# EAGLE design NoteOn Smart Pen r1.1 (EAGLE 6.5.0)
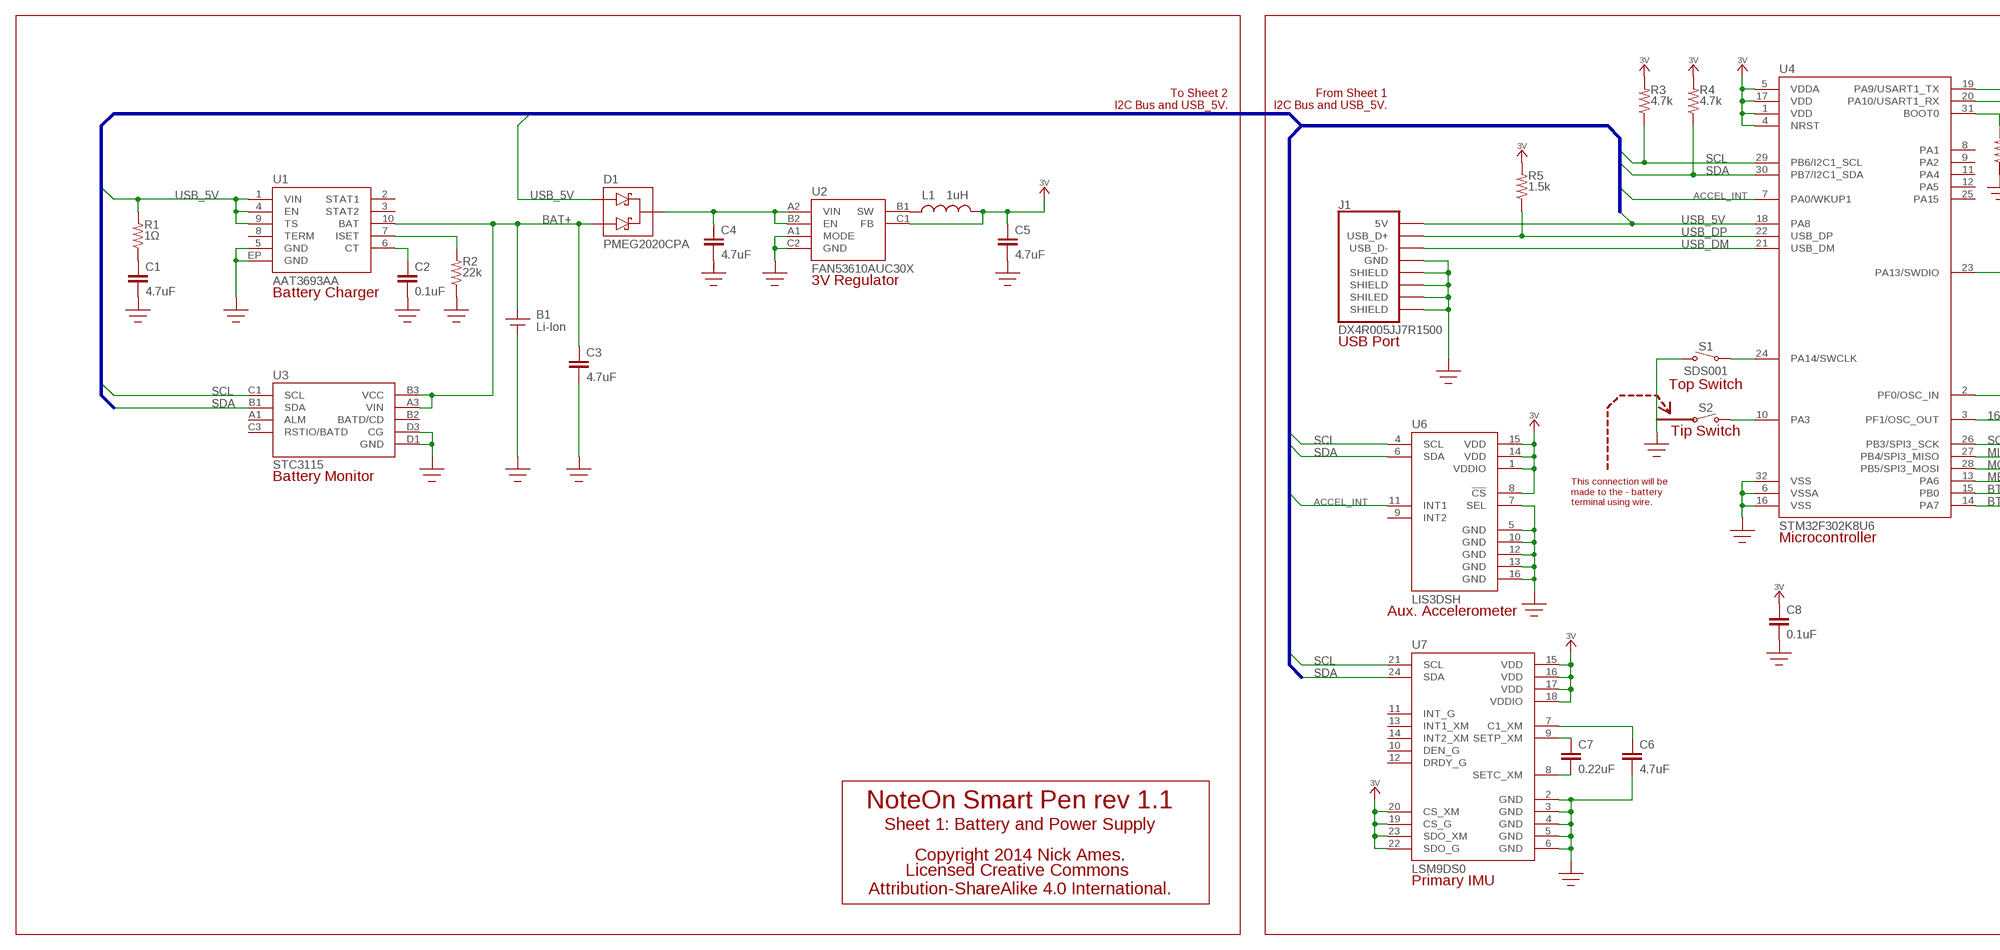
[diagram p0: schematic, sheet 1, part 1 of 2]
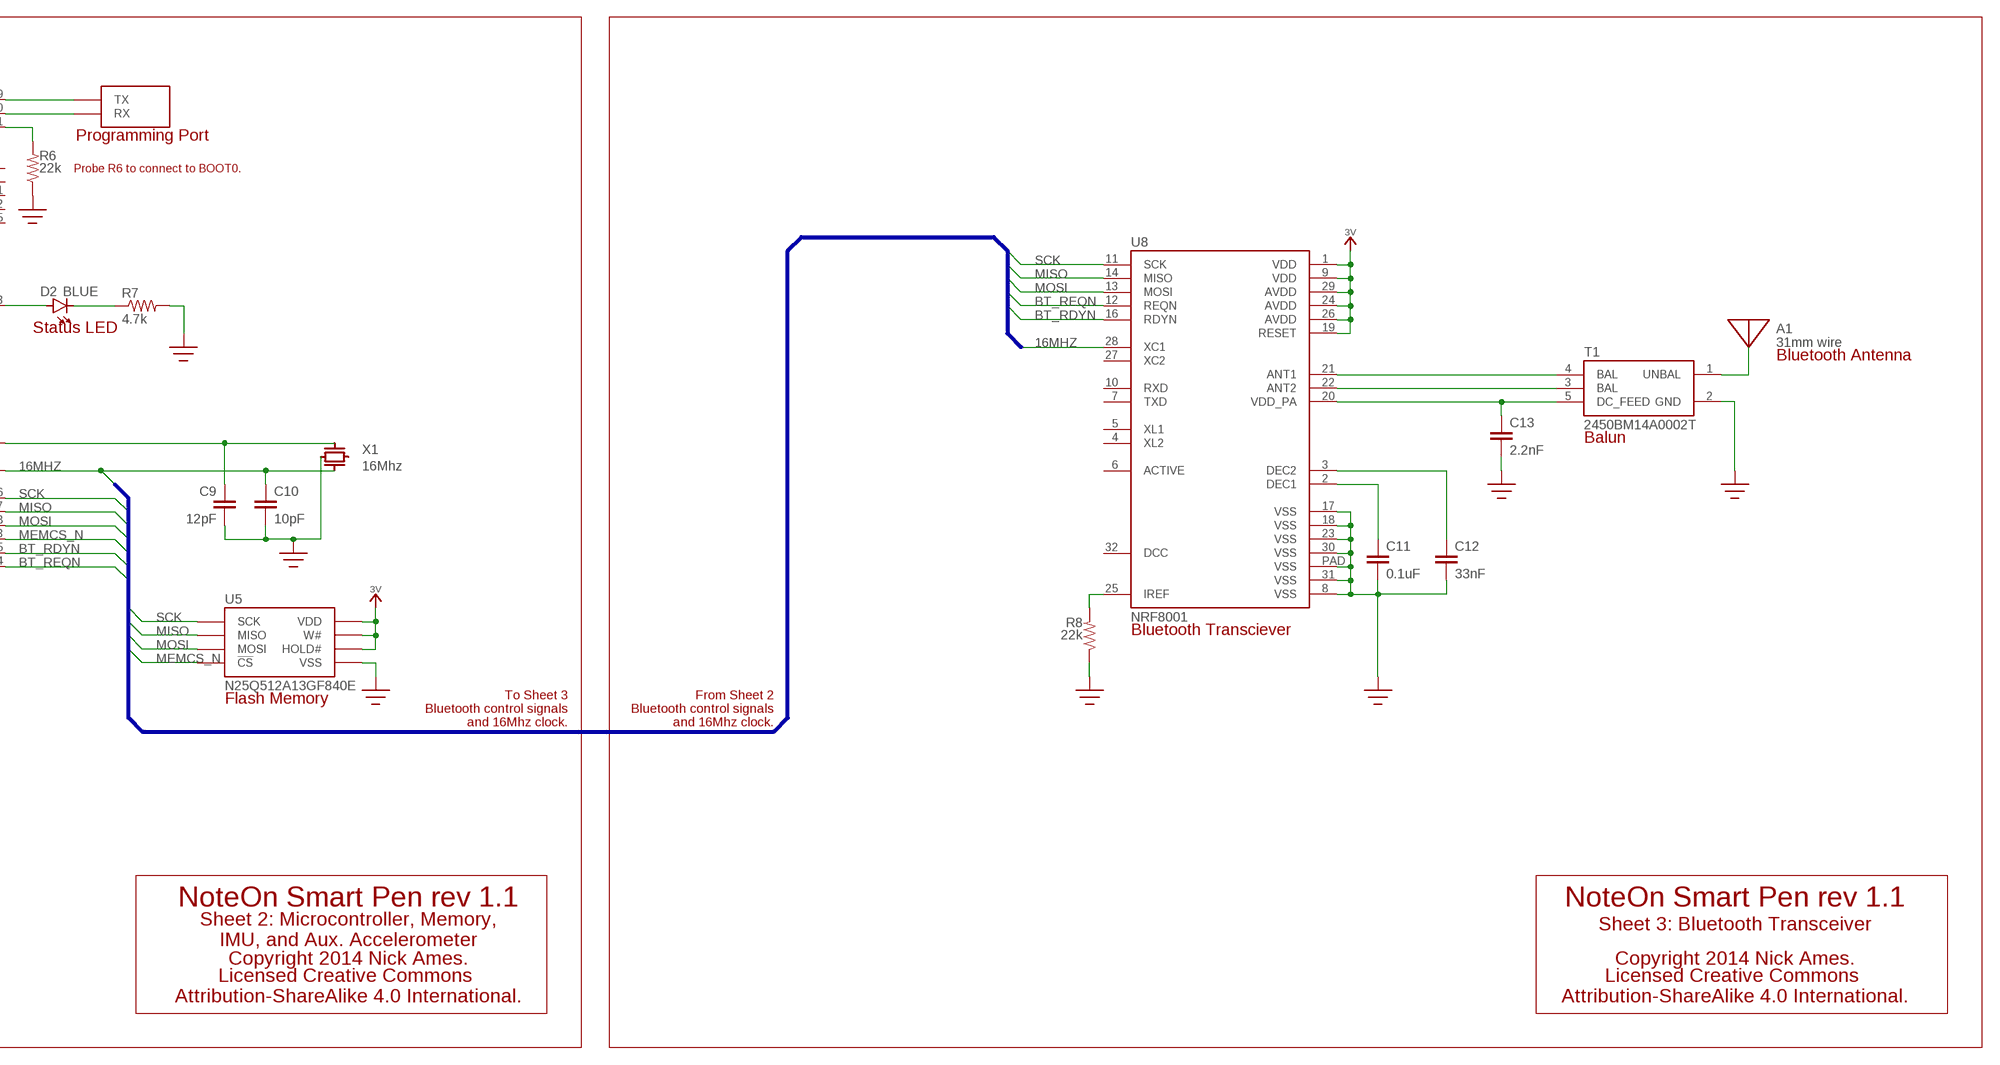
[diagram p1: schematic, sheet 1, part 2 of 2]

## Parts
A1  31mm wire  ANTENNA-WIRE  [WIRE-1]
B1  Li-Ion  BATTERY-1CELL  [BATTERY-WIRETERM]
C1  4.7uF  CAP402  [0402]
C2  0.1uF  CAP402  [0402]
C3  4.7uF  CAP402  [0402]
C4  4.7uF  CAP402  [0402]
C5  4.7uF  CAP402  [0402]
C6  4.7uF  CAP402  [0402]
C7  0.22uF  CAP402  [0402]
C8  0.1uF  CAP402  [0402]
C9  12pF  CAP402  [0402]
C10  10pF  CAP402  [0402]
C11  0.1uF  CAP402  [0402]
C12  33nF  CAP402  [0402]
C13  2.2nF  CAP402  [0402]
D1  PMEG2020CPA  [SOT1061]
D2  BLUE  LED0603  [LED-0603]
J1  DX4R005JJ7R1500  USB_CONNECTORMICRO-MID-SMD  [DX4R005JJ7R1500]
L1  1uH  INDUCTOR805  [0805-IND]
R1  1Ω  RESISTOR402  [0402]
R2  22k  RESISTOR402  [0402]
R3  4.7k  RESISTOR402  [0402]
R4  4.7k  RESISTOR402  [0402]
R5  1.5k  RESISTOR402  [0402]
R6  22k  RESISTOR402  [0402]
R7  4.7k  RESISTOR402  [0402]
R8  22k  RESISTOR402  [0402]
S1  SDS001  SWITCH-SPSTSDS001  [SDS001R]
S2  SWITCH-SPST-OFFBOARD  [TESTPOINT]
T1  2450BM14A0002T  [JOHNASON_BALUN]
U1  AAT3693AA  AAT3693  [TDFN-10]
U2  FAN53610AUC30X  FAN53600  [WLCSP-6]
U3  STC3115  [CSP-10]
U4  STM32F302K8U6  STM32F302K8U6QFN-32  [QFN-32-0.5]
U5  N25Q512A13GF840E  [V-PDFN-8]
U6  LIS3DSH  [LGA-16]
U7  LSM9DS0  [LGA-24]
U8  NRF8001  [QFN-32-0.5-EP]
U$20  STM-PROGPORT  [STM-PROGPORT]
X1  16Mhz  CRYSTAL-2GND  [TXC-8Y]

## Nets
3V: C5.1 C8.1 L1.P$2 R3.2 R4.2 R5.2 U2.C1(FB) U4.1(VDD) U4.4(NRST) U4.5(VDDA) U4.17(VDD) U5.3(W#) U5.7(HOLD#) U5.8(VDD) U6.1(VDDIO) U6.8(!CS!) U6.14(VDD) U6.15(VDD) U7.15(VDD) U7.16(VDD) U7.17(VDD) U7.18(VDDIO) U7.19(CS_G) U7.20(CS_XM) U7.22(SDO_G) U7.23(SDO_XM) U8.1(VDD) U8.9(VDD) U8.19(RESET) U8.24(AVDD) U8.26(AVDD) U8.29(AVDD)
16MHZ: C10.1 U4.3(PF1/OSC_OUT) U8.28(XC1) X1.X2(XTAL2)
ACCEL_INT: U4.7(PA0/WKUP1) U6.11(INT1)
BAT+: B1.+ C3.1 D1.A2 U1.10(BAT) U3.A3(VIN) U3.B3(VCC)
BOOT0: R6.2 U4.31(BOOT0)
BT_RDYN: U4.15(PB0) U8.16(RDYN)
BT_REQN: U4.14(PA7) U8.12(REQN)
GND: B1.- C1.2 C2.2 C3.2 C4.2 C5.2 C6.2 C8.2 C9.2 C10.2 C11.2 C12.2 C13.2 J1.5(GND) J1.SHIELD1(SHIELD) J1.SHIELD2(SHIELD) J1.SHIELD3(SHIELD) J1.SHIELD4(SHILED) R2.1 R6.1 R7.2 R8.1 S1.2 T1.2(GND) U1.5(GND) U1.EP(GND) U2.A1(MODE) U2.C2(GND) U3.D1(GND) U3.D3(CG) U4.6(VSSA) U4.16(VSS) U4.32(VSS) U5.4(VSS) U6.5(GND) U6.7(SEL) U6.10(GND) U6.12(GND) U6.13(GND) U6.16(GND) U7.2(GND) U7.3(GND) U7.4(GND) U7.5(GND) U7.6(GND) U8.8(VSS) U8.17(VSS) U8.18(VSS) U8.23(VSS) U8.30(VSS) U8.31(VSS) U8.PAD(VSS) X1.GND2(GND)
MEMCS_N: U4.13(PA6) U5.1(!CS!)
MISO: U4.27(PB4/SPI3_MISO) U5.2(MISO) U8.14(MISO)
MOSI: U4.28(PB5/SPI3_MOSI) U5.5(MOSI) U8.13(MOSI)
N$1: C1.1 R1.1
N$2: C9.1 U4.2(PF0/OSC_IN) X1.X1(XTAL1)
N$3: C2.1 U1.6(CT)
N$4: S1.1 U4.24(PA14/SWCLK)
N$5: D2.C R7.1
N$6: D2.A U4.23(PA13/SWDIO)
N$7: R2.2 U1.7(ISET)
N$8: L1.P$1 U2.B1(SW)
N$9: S2.1 U4.10(PA3)
N$10: R8.2 U8.25(IREF)
N$14: T1.4(BAL) U8.21(ANT1)
N$15: C7.1 U7.9(SETP_XM)
N$16: C7.2 U7.8(SETC_XM)
N$17: C6.1 U7.7(C1_XM)
N$18: T1.3(BAL) U8.22(ANT2)
N$19: C13.1 T1.5(DC_FEED) U8.20(VDD_PA)
N$20: C11.1 U8.2(DEC1)
N$21: C12.1 U8.3(DEC2)
N$22: A1.1(FEED) T1.1(UNBAL)
REG_VIN: C4.1 D1.C U2.A2(VIN) U2.B2(EN)
RX: U4.20(PA10/USART1_RX) U$20.RX
SCK: U4.26(PB3/SPI3_SCK) U5.6(SCK) U8.11(SCK)
SCL: R3.1 U3.C1(SCL) U4.29(PB6/I2C1_SCL) U6.4(SCL) U7.21(SCL)
SDA: R4.1 U3.B1(SDA) U4.30(PB7/I2C1_SDA) U6.6(SDA) U7.24(SDA)
TX: U4.19(PA9/USART1_TX) U$20.TX
USB_5V: D1.A1 J1.1(5V) R1.2 U1.1(VIN) U1.4(EN) U1.9(TS) U4.18(PA8)
USB_DM: J1.2(USB_D-) U4.21(USB_DM)
USB_DP: J1.3(USB_D+) R5.1 U4.22(USB_DP)
Unconnected: U1.2(STAT1) U1.3(STAT2) U1.8(TERM) U3.A1(ALM) U3.B2(BATD/CD) U3.C3(RSTIO/BATD) U4.8(PA1) U4.9(PA2) U4.11(PA4) U4.12(PA5) U4.25(PA15) U6.9(INT2) U7.10(DEN_G) U7.11(INT_G) U7.12(DRDY_G) U7.13(INT1_XM) U7.14(INT2_XM) U8.4(XL2) U8.5(XL1) U8.6(ACTIVE) U8.7(TXD) U8.10(RXD) U8.27(XC2) U8.32(DCC) X1.GND

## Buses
USB_5V,SDA,SCL,ACCEL_INT
SCK,MISO,MOSI,MEMCS_N,16MHZ,BT_REQN,BT_RDYN

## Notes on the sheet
- To Sheet 2
  I2C Bus and USB_5V.
- From Sheet 1
  I2C Bus and USB_5V.
- Programming Port
- Probe R6 to connect to BOOT0.
- 3V Regulator
- Battery Charger | Status LED
- Bluetooth Antenna
- USB Port
- Top Switch
- Balun
- Tip Switch
- Battery Monitor
- This connection will be
  made to the - battery 
  terminal using wire.
- Microcontroller
- Bluetooth Transciever
- Aux. Accelerometer
- To Sheet 3
  Bluetooth control signals
  and 16Mhz clock.
- From Sheet 2
  Bluetooth control signals
  and 16Mhz clock.
- Flash Memory
- NoteOn Smart Pen rev 1.1 | NoteOn Smart Pen rev 1.1 | NoteOn Smart Pen rev 1.1
- Sheet 1: Battery and Power Supply | Sheet 3: Bluetooth Transceiver
- Sheet 2: Microcontroller, Memory,
  IMU, and Aux. Accelerometer
- Copyright 2014 Nick Ames. | Copyright 2014 Nick Ames. | Copyright 2014 Nick Ames.
- Licensed Creative Commons 
  Attribution-ShareAlike 4.0 International.
- Licensed Creative Commons 
  Attribution-ShareAlike 4.0 International.
- Licensed Creative Commons 
  Attribution-ShareAlike 4.0 International.
- Primary IMU

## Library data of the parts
A1 = NA-lib:ANTENNA-WIRE
B1 = NA-lib:BATTERY-1CELL
C1-C13 = NA-lib:CAP: Capacitor
D1 = NA-lib:PMEG2020CPA
D2 = NA-lib:LED: LEDs
J1 = NA-lib:USB_CONNECTOR
L1 = NA-lib:INDUCTOR: Inductors
R1-R8 = NA-lib:RESISTOR: Resistor
S1 = NA-lib:SWITCH-SPST
S2 = NA-lib:SWITCH-SPST-OFFBOARD
T1 = NA-lib:2450BM14A0002T
U1 = NA-lib:AAT3693
U2 = NA-lib:FAN53600
U3 = NA-lib:STC3115
U4 = NA-lib:STM32F302K8U6
U5 = NA-lib:N25Q512A13GF840E
U6 = NA-lib:LIS3DSH
U7 = NA-lib:LSM9DS0
U8 = NA-lib:NRF8001
U$20 = NA-lib:STM-PROGPORT
X1 = NA-lib:CRYSTAL-2GND

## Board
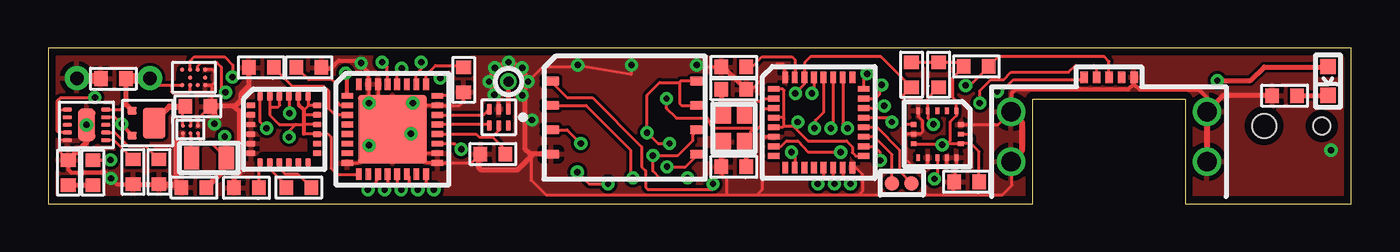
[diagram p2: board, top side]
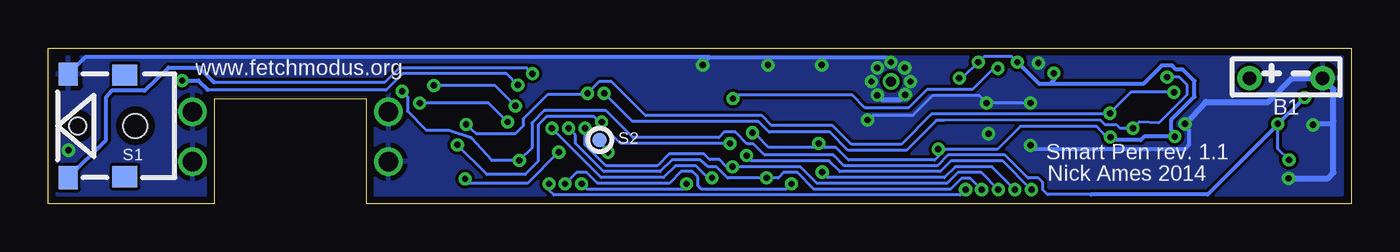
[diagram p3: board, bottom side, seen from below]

Size 67.87 x 8.13 mm. Coordinates in mm from the lower left corner, seen from the top.
Outline: 67.87,0 67.87,8.13 0,8.13 0,0 51.28,0 51.28,5.46 59.21,5.46 59.21,0 67.87,0
Copper layers (1*16): Top 0.0356mm / dielectric 1.5011mm / Bottom 0.0356mm
Design rules "LaenPCBOrder-tented_vias": minimum track width 6mil, minimum drill 13mil, track to track 6mil, track to pad 6mil, pad to pad 6mil, via to via 6mil, smd to smd 6mil, copper to edge 15mil, drill to drill 6mil, minimum pad ring 7mil, minimum via ring 7mil, stop-mask expansion 3mil, vias tented up to drill 25mil, thermal gap 10mil
tRestrict: area 16,3.7 to 16.1,4.1; area 19.7,3.7 to 19.8,4.1; area 11.1,2.5 to 13.7,2.5; area 13.6,2.5 to 13.7,3.4; area 1.4,3.9 to 1.5,4.3; area 2.5,3.9 to 2.6,4.4; area 6.8,6.4 to 7.2,6.8

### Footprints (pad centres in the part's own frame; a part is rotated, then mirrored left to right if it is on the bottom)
WIRE-1 = drill 0.508: 1 0,0
BATTERY-WIRETERM = drill 0.7 pad 1.27: + -1.905,0; - 1.905,0
0402 = smd 0.7 x 0.762: 1 -0.65,0; 2 0.65,0
SOT1061 = smd 0.4 x 0.5: A1 -0.65,0.8; A2 0.65,0.8 | smd 1.6 x 1.2: C 0,-0.35
LED-0603 = smd 0.8 x 0.8: A -0.75,0; C 0.75,0
DX4R005JJ7R1500 = smd 0.4 x 0.6: 1 -1.3,6.096; 2 -0.65,6.096; 3 0,6.096; 4 0.65,6.096; 5 1.3,6.096 | drill 1 pad 1.422: SHIELD1 -5.1,1.7; SHIELD2 -5.1,4.3; SHIELD3 5.1,4.3; SHIELD4 5.1,1.7
0805-IND = smd 0.8 x 1.2: P$1 -0.9,0; P$2 0.9,0
SDS001R = smd 1 x 1.2: 1 1.95,2.7; 2 1.95,-2.7 | smd 1.3 x 1.1: NC -1,2.65; NC2 -1,-2.65 | hole 0.9: 1.45,0 | hole 1.25: -1.55,0
TESTPOINT = smd 0.762 x 0.762: 1 0,0
JOHNASON_BALUN = smd 0.25 x 0.55: 1 0.5,0.425; 2 0,0.425; 3 -0.5,0.425; 4 -0.5,-0.425; 5 0,-0.425; 6 0.5,-0.425
TDFN-10 = smd 0.5 x 0.2: 1 -1,0.8; 2 -1,0.4; 3 -1,0; 4 -1,-0.4; 5 -1,-0.8; 6 1,-0.8; 7 1,-0.4; 8 1,0; 9 1,0.4; 10 1,0.8 | smd 0.9 x 1.7: EP 0,0
WLCSP-6 = smd 0.2 x 0.2: A1 -0.2,0.4; A2 0.2,0.4; B1 -0.2,0; B2 0.2,0; C1 -0.2,-0.4; C2 0.2,-0.4
CSP-10 = smd 0.24 x 0.24: A1 0.4,0.6; A3 -0.4,0.6; B1 0.4,0.2; B2 0,0.2; B3 -0.4,0.2; C1 0.4,-0.2; C3 -0.4,-0.2; D1 0.4,-0.6; D2 0,-0.6; D3 -0.4,-0.6
QFN-32-0.5 = smd 0.6 x 0.3: 1 -2.35,1.75; 2 -2.35,1.25; 3 -2.35,0.75; 4 -2.35,0.25; 5 -2.35,-0.25; 6 -2.35,-0.75; 7 -2.35,-1.25; 8 -2.35,-1.75; 17 2.35,-1.75; 18 2.35,-1.25; 19 2.35,-0.75; 20 2.35,-0.25; 21 2.35,0.25; 22 2.35,0.75; 23 2.35,1.25; 24 2.35,1.75 | smd 0.3 x 0.6: 9 -1.75,-2.35; 10 -1.25,-2.35; 11 -0.75,-2.35; 12 -0.25,-2.35; 13 0.25,-2.35; 14 0.75,-2.35; 15 1.25,-2.35; 16 1.75,-2.35; 25 1.75,2.35; 26 1.25,2.35; 27 0.75,2.35; 28 0.25,2.35; 29 -0.25,2.35; 30 -0.75,2.35; 31 -1.25,2.35; 32 -1.75,2.35
V-PDFN-8 = smd 0.889 x 0.457: 1 -3.835,1.905; 2 -3.835,0.635; 3 -3.835,-0.635; 4 -3.835,-1.905; 5 3.835,-1.905; 6 3.835,-0.635; 7 3.835,0.635; 8 3.835,1.905
LGA-16 = smd 0.356 x 0.254: 1 -1.219,0.996; 2 -1.219,0.498; 3 -1.219,0; 4 -1.219,-0.498; 5 -1.219,-0.996; 9 1.219,-0.996; 10 1.219,-0.498; 11 1.219,0; 12 1.219,0.498; 13 1.219,0.996 | smd 0.254 x 0.356: 6 -0.5,-1.225; 7 0,-1.225; 8 0.5,-1.225; 14 0.5,1.225; 15 0,1.225; 16 -0.5,1.225
LGA-24 = smd 0.45 x 0.3: 1 -1.725,1.25; 2 -1.725,0.75; 3 -1.725,0.25; 4 -1.725,-0.25; 5 -1.725,-0.75; 6 -1.725,-1.25; 13 1.725,-1.25; 14 1.725,-0.75; 15 1.725,-0.25; 16 1.725,0.25; 17 1.725,0.75; 18 1.725,1.25 | smd 0.3 x 0.45: 7 -1.25,-1.725; 8 -0.75,-1.725; 9 -0.25,-1.725; 10 0.25,-1.725; 11 0.75,-1.725; 12 1.25,-1.725; 19 1.25,1.725; 20 0.75,1.725; 21 0.25,1.725; 22 -0.25,1.725; 23 -0.75,1.725; 24 -1.25,1.725
QFN-32-0.5-EP = smd 0.6 x 0.3: 1 -2.35,1.75; 2 -2.35,1.25; 3 -2.35,0.75; 4 -2.35,0.25; 5 -2.35,-0.25; 6 -2.35,-0.75; 7 -2.35,-1.25; 8 -2.35,-1.75; 17 2.35,-1.75; 18 2.35,-1.25; 19 2.35,-0.75; 20 2.35,-0.25; 21 2.35,0.25; 22 2.35,0.75; 23 2.35,1.25; 24 2.35,1.75 | smd 0.3 x 0.6: 9 -1.75,-2.35; 10 -1.25,-2.35; 11 -0.75,-2.35; 12 -0.25,-2.35; 13 0.25,-2.35; 14 0.75,-2.35; 15 1.25,-2.35; 16 1.75,-2.35; 25 1.75,2.35; 26 1.25,2.35; 27 0.75,2.35; 28 0.25,2.35; 29 -0.25,2.35; 30 -0.75,2.35; 31 -1.25,2.35; 32 -1.75,2.35 | smd 3.581 x 3.581: PAD 0,0
STM-PROGPORT = smd 0.762 x 0.762: RX 0,0; TX 0,1.016
TXC-8Y = smd 0.9 x 0.8: GND -0.7,0.55; GND2 0.7,-0.55; X1 -0.7,-0.55; X2 0.7,0.55

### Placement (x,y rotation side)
A1  23.98,6.38 0 top
B1  3.4,6.55 0 bottom
C1  1.05,1.63 90 top
C2  4.43,1.66 270 top
C3  3.4,6.53 180 top
C4  7.8,5.08 0 top
C5  7.61,0.85 180 top
C6  10.34,0.84 180 top
C7  13.06,0.85 180 top
C8  47.83,1.14 180 top
C9  35.71,5.97 0 top
C10  35.71,1.93 180 top
C11  13.59,7.11 0 top
C12  11.1,7.11 180 top
C13  23.16,2.59 180 top
D1  5.18,4.2 90 top
D2  66.65,6.4 270 top
J1  55.24,0.5 0 top
L1  8.38,2.39 0 top
R1  2.34,1.63 90 top
R2  5.78,1.66 90 top
R3  46.38,6.73 90 top
R4  44.96,6.73 90 top
R5  48.34,7.16 180 top
R6  35.71,7.14 0 top
R7  64.39,5.64 180 top
R8  21.64,6.46 90 top
S1  64.87,4.06 180 bottom
S2  39.14,3.33 0 bottom
T1  23.47,4.51 0 top
U1  2.01,4.11 0 top
U2  7.42,3.87 90 top
U3  7.59,6.59 90 top
U4  40.13,4.24 0 top
U5  30.02,4.5 0 top
U6  46.3,3.63 270 top
U7  12.29,3.89 0 top
U8  17.93,3.89 0 top
U$20  44.96,1.07 90 top
X1  35.71,3.94 270 top

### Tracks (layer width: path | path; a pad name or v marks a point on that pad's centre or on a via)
3V  (via drill 0.33 pad 0.69)
  Top 0.152: U2.C1 7.82,3.44 8.03,3.23 8.44,3.23 9.1,2.57 L1.P$2 | U8.29 17.66,7.13 v17.4,7.39 | 19.15,6.27 19.15,6.76 19.43,7.04 v19.43,7.39 | 13.34,3.66 13.36,3.64 U7.15 14.58,3.64 14.73,3.48 14.73,1.85 15.06,1.52 16.17,1.52 U8.9 | 13.06,5.16 13.06,5.6 U7.20 | U7.19 13.54,5.08 | 13.54,5.08 13.34,4.88 | U7.18 13.59,5.14 13.54,5.08 | U7.17 13.42,4.64 13.34,4.72 | U7.16 13.36,4.14 13.34,4.12 | U7.23 11.54,5.12 | 11.54,5.12 11.61,5.05 11.99,5.05 12.06,5.13 12.06,5.59 U7.22 | 11.54,5.12 11.54,4.64 12.04,4.14 12.9,4.14 | 12.9,4.14 13.26,4.14 13.34,4.06 | v20.42,6.55 20.7,6.55 20.93,6.33 20.93,5.71 20.85,5.64 U8.24 | v12.55,3.48 12.55,3.79 12.9,4.14 | U8.19 21.15,3.14 v21.51,2.85 | U5.8 32.94,6.4 32.89,6.35 | 32.89,6.35 32.89,5.23 32.99,5.13 U5.7 | 32.89,6.35 32.87,6.33 31.85,6.33 31.19,5.66 v31.19,3.71 31.75,3.15 v32.36,3.15 | U5.3 27.03,3.86 v27.74,3.15 | U4.5 38.26,3.99 38.33,4.06 | 38.33,4.06 38.33,4.45 | 38.33,4.45 38.28,4.5 U4.4 | 38.33,4.45 38.33,5.92 38.25,5.99 U4.1 | U4.17 42.06,2.49 41.88,2.67 41.88,2.97 41.58,3.28 39.57,3.28 38.79,4.06 | 38.33,4.06 38.79,4.06 | R4.2 R3.2 47.47,7.38 R5.2 47.12,6.59 47.12,5.54 47.3,5.35 U6.1 47.3,4.6 46.97,4.27 46.97,3.28 46.84,3.15 | 38.79,4.06 38.84,4.06 v39.04,4.27 | U6.15 47.9,3.63 48.08,3.45 48.08,3.28 48.01,3.2 | 48.01,3.2 47.95,3.15 47.55,3.15 U6.14 47.51,3.15 46.84,3.15 | U6.8 46.5,3.13 v46.56,3.07 46.76,3.07 46.84,3.15 | C8.1 48.48,2.73 48.01,3.2
  Top 0.203: 13.34,3.66 13.34,4.06 13.34,4.12 13.34,4.72 13.34,4.88 13.06,5.16 | U8.1 15.58,6.72 v15.49,6.81
  Top 0.254: 19.15,6.27 U8.26
  Top 0.305: C5.1 9.1,1.69 9.1,2.57 | 9.3,2.4 L1.P$2 9.28,3.42 v9.2,3.5
  Bottom 0.152: v20.42,6.55 20.3,6.55 v19.43,7.39 19.15,7.67 17.68,7.67 v17.4,7.39 | v12.55,3.48 12.75,3.48 13.26,4.04 17.25,4.04 18.44,2.85 21.13,2.85 | v21.51,2.85 21.13,2.85 | 21.13,2.85 21.69,2.29 26.19,2.29 26.85,2.95 27.61,2.95 27.61,3.02 v27.74,3.15 27.74,3.1 27.89,2.95 30.35,2.95 30.94,3.53 31.19,3.53 v31.19,3.71 | v32.36,3.15 38.05,3.15 39.12,4.22 | 39.12,4.22 39.45,4.55 41.91,4.55 42.34,4.12 42.34,2.21 43.03,1.52 45.01,1.52 v46.56,3.07 | v39.04,4.27 39.06,4.27 39.12,4.22
  Bottom 0.203: v12.55,3.48 12.39,3.33 10.97,3.33 10.79,3.5 v9.2,3.5 9.2,3.66 9.37,3.83 9.37,4.39 8.18,5.59 8.18,6.4 8.79,7.01 9.14,7.01 9.35,7.21 9.88,7.21 10.85,6.25 15.7,6.25 | 15.7,6.25 16.26,6.25 v17.4,7.39 | v15.49,6.81 15.49,6.45 15.7,6.25
16MHZ  (via drill 0.33 pad 0.69)
  Top 0.152: 36.56,3.24 X1.X2 36.55,3.52 36.55,3.73 36.75,3.94 | U8.28 18.18,6.88 v18.41,7.06 | 36.75,3.94 34.62,3.94 34.34,4.47 32.72,4.47 32.21,4.98 v32.21,5.49 | 36.75,3.94 36.96,3.94 37.11,4.09 37.11,4.83 37.26,4.98 37.77,4.98 U4.3
  Top 0.254: C10.1 36.36,3.14 X1.X2
  Bottom 0.152: v18.41,7.06 18.64,7.06 19.74,5.97 22.1,5.97 23.06,5 25.32,5 25.98,5.66 32.03,5.66 v32.21,5.49
ACCEL_INT  (via drill 0.33 pad 0.69)
  Top 0.152: U4.7 38.17,2.99 38.46,3.28 39.04,3.28 39.57,2.69 v41.27,2.69 | U6.11 46.3,1.45 v46.15,1.29
  Bottom 0.152: v41.27,2.69 42.9,1.07 45.92,1.07 v46.15,1.29
BAT+
  Top 0.152: U1.10 3.77,4.93 4.05,5.21 | B1.+ 5.67,6.19 6.44,6.19 | 6.44,6.19 U3.A3 | 6.44,6.19 6.44,5.83 6.5,5.77 7.29,5.77 7.39,5.87 U3.B3
  Top 0.254: C3.1 4.05,5.21 D1.A2
  Top 0.61: C3.1 B1.+
BOOT0
  Top 0.152: R6.2 36.65,7.14 37.19,7.67 38.73,7.67 38.89,7.52 U4.31
BT_RDYN  (via drill 0.33 pad 0.69)
  Top 0.152: U8.16 19.68,1.15 v20.09,0.74 | U4.15 41.38,1.44 v41.78,1.04
  Bottom 0.152: v20.09,0.74 20.37,0.46 41.53,0.46 41.78,0.71 v41.78,1.04
BT_REQN  (via drill 0.33 pad 0.69)
  Top 0.152: U8.12 17.68,0.89 v17.53,0.74 | v27.56,1.65 28.17,1.04 v29.16,1.04 | U4.14 40.88,1.1 v40.95,1.04
  Bottom 0.152: v17.53,0.74 18.72,1.93 20.62,1.93 21.18,1.37 27.28,1.37 v27.56,1.65 | v29.16,1.04 29.44,0.76 33.86,0.76 34.04,0.94 34.04,1.4 34.31,1.68 34.9,1.68 35.51,1.07 39.27,1.07 39.83,1.63 40.36,1.63 v40.95,1.04
GND  (via drill 0.33 pad 0.69)
  Top 0.152: U1.5 0.61,3.33 0.56,3.28 0.56,2.77 C1.2 | U3.D3 8.53,6.19 | 8.53,6.19 8.71,6.38 8.71,6.83 8.55,6.99 U3.D1 | 8.53,6.19 8.53,5.26 C4.2 8.42,5.05 7.82,4.45 U2.C2 | U2.A1 7.02,3.38 6.96,3.33 6.76,3.33 6.66,3.23 | 8.66,4.8 8.66,4.75 8.76,4.65 | U7.2 10.56,4.65 9.98,4.65 | U7.4 10.55,3.66 9.98,3.66 | 10.55,3.15 U7.5 9.99,3.14 9.98,3.12 | U7.6 10.03,2.64 9.98,2.59 | U7.3 9.99,4.14 9.98,4.14 | U8.30 17.18,5.42 | U8.8 16.18,2.14 U8.PAD | 19.36,5.14 U8.23 21.42,5.14 21.64,5.36 R8.1 | U8.18 19.18,2.64 U8.PAD | U8.PAD 19.68,2.14 U8.17 22.06,2.14 22.4,2.48 C13.2 | 17.17,5.41 17.12,5.46 16.69,5.46 16.68,5.47 U8.31 16.68,6.84 | 14.29,7.06 C11.2 | 17.37,3.89 U8.PAD | 18.95,3.25 18.75,3.45 18.31,3.89 U8.PAD | v25.2,4.37 24.82,4.7 24.82,5.51 | T1.2 23.47,5.46 v23.24,5.69 | v16.31,7.34 16.24,7.28 | 25.15,2.59 25.15,1.25 25.93,0.46 35.38,0.46 | 35.38,0.46 36.91,0.46 | 36.91,0.46 42.22,0.46 | C10.2 35.06,1.56 35.33,1.29 35.33,0.51 35.38,0.46 | X1.GND2 35.16,3.54 35.31,3.54 | R6.1 33.88,7.14 v33.78,7.24 | U4.6 37.33,3.49 37.19,3.35 37.19,0.74 36.91,0.46 | 42.22,0.46 45.77,0.46 | 45.77,0.46 47.12,0.46 | 47.12,0.46 49.68,0.46 50.19,0.96 50.19,2.15 J1.SHIELD1 | 45.8,2.4 U6.10 45.81,2.14 45.57,1.91 | U6.13 47.3,2.04 47.22,1.91 | 47.22,1.91 46.89,1.91 46.79,2.01 46.8,2.02 U6.12 46.79,2.4 | 45.57,1.91 45.06,1.91 44.65,2.34 44.65,3.53 44.76,3.63 U6.7 45.41,3.63 45.52,3.73 45.52,4.34 45.31,4.55 U6.5 | U4.16 42.05,1.89 42.42,1.52 42.42,0.66 42.22,0.46 | C9.2 36.63,5.97 37.95,7.29 38.28,7.29 38.38,7.19 U4.32 | 47.22,1.91 47.22,1.18 C8.2 47.12,1.08 47.12,0.46 | 45.57,1.91 45.57,0.64 45.77,0.46 | U6.16 49.48,4.13 J1.SHIELD2 | v24.99,6.38 25.78,7.16 27.23,7.16 v27.58,7.24 30.38,6.76 v30.38,7.24
  Top 0.203: C1.2 1.05,1.79 1.22,1.63 2.97,1.63 v3.28,1.32 3.58,1.02 C2.2 | 14.29,7.06 14.73,7.06 15.14,7.47 16.05,7.47 16.24,7.28 16.68,6.84 | v16.71,3.05 18.09,3.05 v18.9,3.66 18.85,3.56 18.75,3.45 | J1.5 56.55,6.25 | 56.55,6.25 56.24,5.94 50.37,5.94 50.16,5.74 50.16,4.82 J1.SHIELD2 | 56.55,6.25 56.85,5.94 59.92,5.94 60.35,5.51 J1.SHIELD3
  Top 0.254: C2.2 R2.1 | U1.EP 2.01,4.52 1.96,4.57 | 6.66,3.23 6.66,1.15 C5.2 | C6.2 9.69,1.31 9.98,1.6 9.98,2.59 9.98,3.12 9.98,3.66 9.98,4.14 9.98,4.65 9.98,4.78 9.7,5.05 | 9.7,5.05 9.65,5.11 8.47,5.11 C4.2 | C12.2 10.45,6.13 10.03,5.71 10.03,5.38 9.7,5.05 | U8.30 | 17.18,5.42 17.17,5.41 17.17,4.65 U8.PAD 19.15,5.11 19.33,5.11 19.36,5.14 | U5.4 25.27,2.59 | 25.27,2.59 25.15,2.59 25.09,2.59 24.84,2.85 24.84,5.49 24.82,5.51 24.69,5.64 v24.69,5.66 v24.99,6.38 v24.69,7.09 v23.98,7.39 v23.27,7.09 v22.96,6.38 v23.24,5.69 | 22.4,2.48 22.4,1.93 22.55,1.78 24.46,1.78 25.27,2.59 | C10.2 35.06,3.14 X1.GND2 | R6.1 35.17,7.14 C9.2 36.26,5.84 | R7.2 61.18,5.64 J1.SHIELD3
  Top 0.305: C1.2 2.01,3.23 U1.EP | R2.1 6.79,1.01 C5.2 | 8.42,5.05 8.66,4.8 v8.66,4.17 | J1.SHIELD3 J1.SHIELD4 | J1.SHIELD2 50.16,4.8 50.7,4.27 50.7,2.75 J1.SHIELD1
  Top 0.61: C3.2 B1.-
  Bottom 0.152: 0.94,4.29 0.94,4.22 0.99,4.17 | v25.2,4.37 24.89,4.62 22.84,4.62 21.79,5.66 19.41,5.66 v19,5.26 v16.71,5.26 | v33.78,7.24 33.43,7.64
  Bottom 0.203: v8.66,4.17 8.66,4.06 8.46,3.86 8.46,3.07 8.69,2.85 16.51,2.85 v16.71,3.05 | v23.98,7.39 24.23,7.64 33.43,7.64 65.94,7.64 S1.2
  Bottom 0.254: 0.99,4.17 1.96,4.17 U1.EP | v23.24,5.69 23.52,5.41 24.43,5.41 v24.69,5.66
  Bottom 0.305: v3.28,1.32 1.25,1.32 0.94,1.63 0.94,4.29 0.94,5.97 B1.- 3.1,6.55 4.34,5.31 7.59,5.31 v8.66,4.17
  other vias: 2.01,4.11 66.8,2.79
  pour Top (isolate 0.152): 0.46,0.46 0.46,7.67 67.41,7.67 67.41,0.46
  pour Bottom (isolate 0.152): 0.46,0.46 0.46,7.67 67.41,7.67 67.41,0.46
MEMCS_N  (via drill 0.33 pad 0.69)
  Top 0.152: v34.62,1.04 34.62,0.76 31.22,0.76 31.11,0.86 31.11,1.73 30.91,1.93 30.91,2.97 28.35,5.54 27.03,5.54 26.19,6.38 U5.1 | U4.13 40.38,1.34 v40.08,1.04
  Bottom 0.152: v34.62,1.04 34.62,0.76 39.8,0.76 v40.08,1.04
MISO  (via drill 0.33 pad 0.69)
  Top 0.152: U8.14 18.8,1.42 18.8,1.14 19.2,0.74 v19.25,0.74 | U5.2 28.02,5.13 30.33,2.82 30.33,1.5 v30.45,1.35 | U4.27 40.88,4.1 v40.77,3.94
  Bottom 0.152: v19.25,0.74 19.84,1.32 20.32,1.32 20.88,0.76 27.99,0.76 28.85,1.63 29.57,1.63 29.84,1.35 v30.45,1.35 32.49,1.35 33.07,1.93 33.48,1.93 33.88,2.29 35.38,2.29 35.99,1.68 38.94,1.68 40.41,3.15 40.41,3.58 v40.77,3.94
MOSI  (via drill 0.33 pad 0.69)
  Top 0.152: U8.13 18.18,0.94 v18.39,0.74 | U4.28 40.38,4.77 39.95,4.34 39.95,4.17 v39.9,3.94 | v32.23,1.93 33.2,1.93 U5.5
  Bottom 0.152: v18.39,0.74 19.28,1.63 20.5,1.63 21.06,1.07 27.84,1.07 28.7,1.93 v32.23,1.93 32.54,1.93 32.92,2.31 33.43,2.31 33.71,2.59 35.53,2.59 36.14,1.98 38.81,1.98 39.9,3.07 v39.9,3.94
N$1
  Top 0.254: C1.1 R1.1
N$2
  Top 0.152: 35.06,4.8 35.06,4.59 | 35.06,5.28 35.09,5.36 37.11,5.36 37.24,5.49 U4.2
  Top 0.254: X1.X1 35.06,4.74 35.06,4.8 35.06,5.28 C9.1
N$3
  Top 0.152: C2.1 3.42,3.33 U1.6
N$4  (via drill 0.33 pad 0.69)
  Top 0.152: U4.24 42.48,6.62 v42.65,6.78
  Bottom 0.152: 59.21,6.33 50.34,6.33 49.58,7.09 42.95,7.09 v42.65,6.78
  Bottom 0.203: S1.1 64.85,3.34 64.85,5.56 64.54,5.89 62.84,5.89 61.59,7.11 59.99,7.11 59.21,6.33
N$5
  Top 0.254: R7.1 66.64,5.64 D2.C
N$6  (via drill 0.33 pad 0.69)
  Top 0.152: U4.23 43.08,5.49 43.31,5.71 43.31,6.1 v43.41,6.2
  Top 0.254: v60.88,6.43 62.61,6.43 63.32,7.14 66.64,7.14 D2.A
  Bottom 0.152: 59.56,5.94 59.54,5.92 50.27,5.92 49.4,6.78 43.99,6.78 v43.41,6.2
  Bottom 0.203: v60.88,6.43 60.05,6.43 59.56,5.94
N$7
  Top 0.152: U1.7 3.46,3.73 4.17,3.02 5.07,3.02 R2.2
N$8
  Top 0.152: U2.B1 7.42,2.45 L1.P$1
N$9  (via drill 0.33 pad 0.69)
  Top 0.152: v38.71,2.69 38.88,2.42 U4.10
  Bottom 0.152: S2.1 39.14,3.23 v38.71,2.69
N$10
  Top 0.152: 21.54,7.39 R8.2 21.59,7.21 20.17,7.21 19.68,6.73 U8.25
N$14
  Top 0.152: T1.4 22.92,4.14 U8.21
N$15
  Top 0.152: U7.9 12.04,1.85 12.34,1.55 13.01,1.55 C7.1
N$16
  Top 0.152: C7.2 12.41,0.95 11.54,1.82 U7.8
N$17
  Top 0.152: C6.1 10.99,2.1 U7.7
N$18
  Top 0.152: U8.22 22.67,4.64 T1.3
N$19
  Top 0.152: U8.20 22.3,3.63 22.45,3.48 23.14,3.48 | 23.14,3.48 23.47,3.81 T1.5 | 23.14,3.48 23.82,2.8 C13.1
N$20
  Top 0.152: U8.2 15.21,5.14 15.04,5.33 15.04,6.22 14.78,6.48 13.57,6.48 C11.1
N$21
  Top 0.152: U8.3 14.95,4.64 14.63,4.95 14.63,5.87 14.38,6.12 12.74,6.12 C12.1
N$22
  Top 0.152: T1.1
  Top 0.254: T1.1 A1.1
REG_VIN
  Top 0.152: U2.A2 7.02,4.46 | 7.02,4.46 7.02,4.95 C4.1 | 7.02,4.46 7.36,4.46 7.42,4.39 U2.B2
  Top 0.305: D1.C 5.53,4.29 6.33,5.08 C4.1
RX
  Top 0.152: U4.20 43.15,3.99 44.32,2.82 44.32,1.7 U$20.RX
SCK  (via drill 0.33 pad 0.69)
  Top 0.152: 16.66,0.76 v16.66,0.74 16.69,0.74 17.09,1.14 17.09,1.22 17.18,1.31 U8.11 | v33.3,1.35 31.85,1.35 31.5,1.7 v31.5,2.52 32.79,2.52 33.58,3.3 33.58,3.58 U5.6 | U4.26 41.38,4.19 v41.63,3.94
  Bottom 0.152: v16.66,0.74 18.16,2.23 20.85,2.23 21.41,1.68 26.64,1.68 27.2,2.23 31.27,2.23 31.5,2.46 v31.5,2.52 31.5,2.77 | v33.3,1.35 33.5,1.35 34.14,1.98 35.2,1.98 35.81,1.37 39.06,1.37 v41.63,3.94
SCL  (via drill 0.33 pad 0.69)
  Top 0.152: U3.C1 7.79,7.18 7.98,7.37 8.79,7.37 9.02,7.14 9.02,6.04 v9.25,5.82 | v12.57,4.72 12.57,5.58 U7.21 | R3.1 45.81,5.51 U6.4 45.81,4.49 v46.1,4.14 | U4.29 39.88,5.87 v39.78,5.77
  Bottom 0.152: v9.25,5.82 11.48,5.82 v12.57,4.72 12.62,4.67 21.87,4.67 23.44,3.1 26.04,3.1 27.03,4.09 30.2,4.09 30.68,4.6 36.75,4.6 38.53,6.38 39.17,6.38 v39.78,5.77 39.83,5.71 41.83,5.71 43.1,4.45 43.1,4.09 43.54,3.66 45.57,3.66 v46.1,4.14
SDA  (via drill 0.33 pad 0.69)
  Top 0.152: U3.B1 7.39,7.45 7.62,7.67 9.2,7.67 9.63,7.24 9.63,6.58 v9.6,6.6 | v11.38,3.94 11.04,4.27 U7.24 | U6.6 44.66,4.13 44.55,4.24 44.55,5.67 R4.1 44.95,6.08 43.36,7.67 39.7,7.67 39.4,7.37 39.4,6.61 | 39.4,6.61 U4.30 | 39.4,6.61 39.4,6.25 v38.91,5.77
  Bottom 0.152: v9.6,6.6 8.97,6.6 8.59,6.22 8.59,5.66 10.03,4.22 11.05,4.27 v11.38,3.94 12.04,3.94 12.22,4.12 12.83,4.12 13.08,4.37 21.21,4.34 21.61,4.34 23.16,2.79 26.21,2.79 27.15,3.73 30.33,3.73 30.89,4.29 37.44,4.29 v38.91,5.77
TX
  Top 0.152: U4.19 42.49,3.48 43.03,3.48 43.94,2.56 U$20.TX
USB_5V  (via drill 0.33 pad 0.69)
  Top 0.152: U1.4 0.59,3.73 0.48,3.79 0.48,4.78 | 0.48,4.78 0.66,4.9 U1.1 | 0.48,4.78 0.48,5.36 0.69,5.54 v2.44,5.54 | U1.9 3.47,4.53 3.67,4.33 v3.83,4.17 | R1.2 3.11,2.28 v3.25,2.29 | U4.18 43.01,2.99 43.31,2.69 43.31,2.29 v43.33,2.26 | v49.43,5.87 49.66,5.87 50.27,6.48 53.83,6.48 J1.1
  Top 0.203: v3.83,4.17 3.83,4.12 D1.A1
  Bottom 0.152: v3.25,2.29 3.83,2.87 3.83,4.14 v3.83,4.17 | v2.44,5.54 2.62,5.36 | 13.56,0.48 15.82,0.48 16.08,0.74 16.08,1.12 16.31,1.35 16.84,1.35 18.03,2.54 21.01,2.54 21.57,1.98 26.42,1.98 26.98,2.54 30.56,2.54 31.14,3.12 31.47,3.12 32.08,3.73 32.66,3.73 32.94,3.45 37.41,3.45 38.81,4.85 42.04,4.85 42.67,4.22 42.67,2.92 v43.33,2.26 44.76,2.26 45.82,3.43 47.02,3.83 48.16,3.83 49.15,4.83 49.15,5.59 v49.43,5.87
  Bottom 0.203: v2.44,5.54 2.62,5.36 v3.83,4.17 | 3.83,4.14 7.49,0.48 13.56,0.48
USB_DM  (via drill 0.33 pad 0.69)
  Top 0.152: 54.59,6.67 J1.2 54.59,7.06 54.43,7.21 53.49,7.21 53.14,6.86 50.14,6.86 49.76,6.48 49.1,6.48 48.51,5.89 v48.51,5.26 | U4.21 43.72,4.49 v43.94,4.27
  Bottom 0.152: v43.94,4.27 44.93,5.26 v48.51,5.26
USB_DP  (via drill 0.33 pad 0.69)
  Top 0.152: J1.3 55.24,7.42 54.99,7.67 49.49,7.67 R5.1 48,6.17 v47.78,6.17 | U4.22 43.42,4.99 v43.54,5.11
  Bottom 0.152: v43.54,5.11 44.6,6.17 v47.78,6.17

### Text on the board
bPlace: www.fetchmodus.org | Smart Pen rev. 1.1 | Nick Ames 2014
